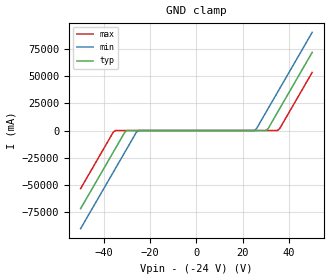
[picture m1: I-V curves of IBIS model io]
| TEXAS INSTRUMENTS INCORPORATED
| 1 Channel Bi-directional ESD-SURGE Protection Device
| Marketing Part #   Voltage Range   Package-type   #pins/pkg drawing
|   TSD24C-Q1   -24V-24V   SOD-323   2/DYF
[IBIS Ver]   4.1
[Comment char]  |_char
[File Name]   tsd24cq1.ibs
[File Rev]   1.0
"[Date]   Dec 20, 2023 "
[Source]   Data created from TI-SPICE simulations at TI-SLL/HVL.
   The following is an IBIS list for the TSD24C.
   Please contact sllibis@ti.com with questions and
   comments concerning SLL IBIS models.
[Notes]
   - New measurements under nominal conditions only.
[Disclaimer]
"| TI and its licensors and suppliers make no warranties, either expressed"
"| or implied, with respect to this  model, including the warranties of "
"| provided solely on an ""as is"" basis. The entire risk as to its quality "
| and performance is with the customer.
[Copyright]
| (C) Copyright 2023 Texas Instruments Incorporated. All rights reserved.
| Component TSD24CQ1_DYF 2-PIN SOD-323
[Component]   TSD24CQ1_DYF
"[Manufacturer]   Texas Instruments, Inc."
[Package]   |2 SOD-323 - DYF package
   typ   min   max
R_pkg   30.0E-03   24.0E-03   36.0E-03
L_pkg   3.8E-10   3.0E-10   4.56E-10
C_pkg   5.7E-13   4.5E-13   6.8E-13
[Pin]   signal_name   model_name   R_pin   L_pin   C_pin
1   IO   io   2.07E-03   2.09E-10   6.95E-14
2   IO   io   2.07E-03   2.09E-10   6.95E-14
3   GND   gnd   2.07E-03   2.09E-10   6.95E-14
| Models and submodels in the file (1): io (Input)
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|   io Model
[Model]   io
Model_type  Input
| variable   typ   min   max
C_comp   4.3pF   3.5pF   5.0pF
[Voltage Range]   48   40   56
[Temperature Range]   27   -55   150
[Power Clamp Reference]   0   0   0
[GND Clamp Reference]   -24   -20   -28
[GND Clamp]
|	Voltage	  I(typ)	  I(min)   I(max)
-50V      -72.2A     -90.7A     -53.7A
-36V      -20.4A     -38.9A     -1.85A
-31V      -1.85A     -20.4A     -5.08nA
-30V      -4.92nA    -16.7A     -4.92nA
-26V      -4.26nA    -1.85A     -4.26nA
-25V      -4.1nA     -4.1nA     -4.1nA
25V       4.1nA      4.1nA      4.1nA
26V       4.26nA     1.85A      4.26nA
30V       4.92nA     16.7A      4.92nA
31V       1.85A      20.4A      5.08nA
36V       20.4A      38.9A      1.85A
50V       72.2A      90.7A      53.7A
[Power Clamp]
|   Voltage   I(typ)   I(min)   I(max)
-24V      0A         0A         0A
0V        0A         0A         0A
24V       0A         0A         0A
